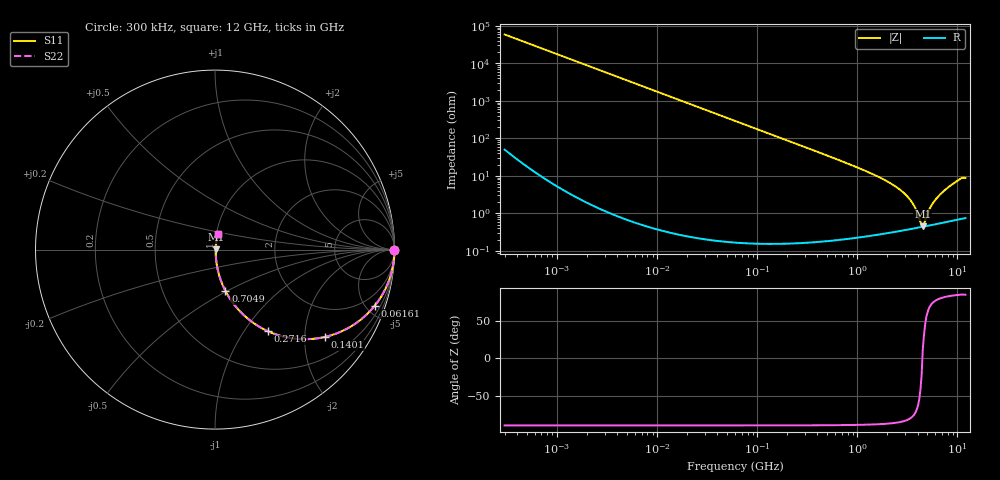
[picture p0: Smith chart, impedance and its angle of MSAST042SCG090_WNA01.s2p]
! MSAST042SCG090_WNA01  S-PARAMETER MODEL  ( General Type )
! Model Generated by TAIYO YUDEN Corporation (http://www.ty-top.com)
! Version 1.0
! TAIYO YUDEN Control No. 150820
! Copyright(c) 2015 TAIYO YUDEN CO.,LTD. All Rights Reserved.
! Product Description (link to TY-COMPAS)
! https://ds.yuden.co.jp/TYCOMPAS/or/detail?pn=MSAST042SCG090BWNA01&u=M
! Products Name : Multilayer Ceramic Capacitors
! Characteristics :
!  Capacitance : 9 pF , Rated Voltage : 25V , TCC : CG / C0G
!  Case Size : 0.4 x 0.2 / 0.016 x 0.008 [mm/inch] , Thickness : 0.2 / 0.008 [mm/inch]
!  (Conditions: Temperature = 25 degC , DC Bias Current/Voltage = 0A / 0V)
! External Node Assignments :
!  1  o---| |---o  2
! GND o---------o GND
! Frequency Range : 0.3MHz  -  12000MHz  [ 401 STEP ]
# MHz S RI R 50
! Freq[MHz].  S11 Real  S11 Imag  S21 Real  S21 Imag  S12 Real  S12 Imag  S22 Real  S22 Imag
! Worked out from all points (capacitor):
!   401 points, 300 kHz to 12 GHz, reference 50 ohm
!   read as one part in series: C = 9.04 pF near 316.3 kHz
!   lowest |Z| = 448 mohm at 4.503 GHz (marker M1)
!   series resonance near 4.464 GHz, so ESL is about 140 pH
!   S11 on the Smith chart (normalised r, x): 300 kHz: open; 61.61 MHz: 1.00, -5.72; 140.1 MHz: 1.00, -2.51; 271.6 MHz: 1.00, -1.29; 704.9 MHz: 1.00, -0.49; 12 GHz: 1.02, +0.18
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0.3  1 -0.0017  4.35e-06 0.0017  4.35e-06 0.0017  1 -0.0017
1.769972  0.9999 -0.01  0.000103 0.01  0.000103 0.01  0.9999 -0.01
10.44266  0.9965 -0.0591  0.00352 0.0591  0.00352 0.0591  0.9965 -0.0591
26.39317  0.978 -0.1465  0.022 0.1465  0.022 0.1465  0.978 -0.1465
60  0.8959 -0.3052  0.1041 0.3052  0.1041 0.3052  0.8959 -0.3052
61.61074  0.8908 -0.3116  0.1092 0.3116  0.1092 0.3116  0.8908 -0.3116
91.67136  0.7865 -0.4093  0.2135 0.4093  0.2135 0.4093  0.7865 -0.4093
140.0606  0.612 -0.4867  0.388 0.4867  0.388 0.4867  0.612 -0.4867
271.6094  0.295 -0.4548  0.705 0.4548  0.705 0.4548  0.295 -0.4548
353.9943  0.1973 -0.3963  0.8027 0.3963  0.8027 0.3963  0.1973 -0.3963
704.9044  0.0577 -0.2292  0.9423 0.2292  0.9423 0.2292  0.0577 -0.2292
2088.533  0.00732 -0.0654  0.9927 0.0654  0.9927 0.0654  0.00732 -0.0654
2722.03  0.00506 -0.0405  0.9949 0.0405  0.9949 0.0405  0.00506 -0.0405
3276.641  0.00435 -0.0248  0.9957 0.0248  0.9957 0.0248  0.00435 -0.0248
3740.715  0.00418 -0.0142  0.9958 0.0142  0.9958 0.0142  0.00418 -0.0142
4270.516  0.00427 -0.00379  0.9957 0.00379  0.9957 0.00379  0.00427 -0.00379
4502.883  0.00437 0.000875  0.9956 -0.000875  0.9956 -0.000875  0.00437 0.000875
4747.894  0.00451 0.00439  0.9955 -0.00439  0.9955 -0.00439  0.00451 0.00439
5420.343  0.00502 0.0142  0.995 -0.0142  0.995 -0.0142  0.00502 0.0142
6524.734  0.00614 0.0285  0.9939 -0.0285  0.9939 -0.0285  0.00614 0.0285
10236.47  0.0126 0.0754  0.9874 -0.0754  0.9874 -0.0754  0.0126 0.0754
12000  0.015 0.0862  0.985 -0.0862  0.985 -0.0862  0.015 0.0862
